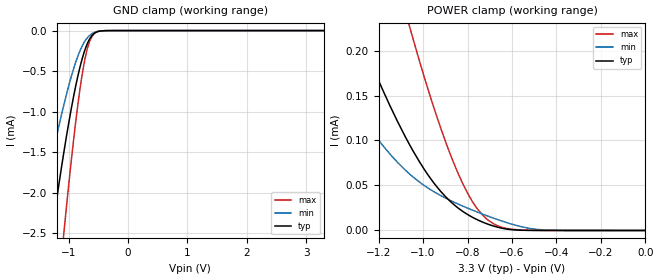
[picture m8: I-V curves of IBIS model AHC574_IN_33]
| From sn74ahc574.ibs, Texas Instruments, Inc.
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[Model]   AHC574_IN_33
Model_type  Input
Vinl = 0.9
Vinh = 2.1
| variable   typ   min   max
C_comp   1.37pF   0.98pF   1.70pF
[Temperature Range]   40   100   -40
| Ambient temperature   25   85   -40
[Voltage range]   3.3   3   3.6
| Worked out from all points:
|   GND clamp passes 1 mA (typ) near -0.97 V on its own axis
|   POWER clamp passes 1 mA (typ) near -2.27 V on its own axis
[GND Clamp]
| AHC574_IN_33
|   Voltage   I(typ)   I(min)   I(max)
-3.3V     -17mA      -11.03mA   -23.02mA
-1.53V    -3.897mA   -2.48mA    -6.164mA
-1.29V    -2.531mA   -1.59mA    -4.125mA
-1.255V   -2.347mA   -1.47mA    -3.84mA
-1.105V   -1.604mA   -983.1uA   -2.663mA
-1.075V   -1.466mA   -892.6uA   -2.438mA
-910mV    -781.9uA   -451.4uA   -1.295mA
-775mV    -351.6uA   -192.7uA   -547.4uA
-680mV    -149.8uA   -83.75uA   -205.8uA
-580mV    -40.35uA   -26.33uA   -44.58uA
-380mV    -1.07uA    -806.4nA   -548.9nA
3.3V      2.685nA    5.487nA    12.92nA
[POWER Clamp]
| AHC574_IN_33
|   Voltage   I(typ)   I(min)   I(max)
-3.3V     2.071mA    1.373mA    3.367mA
-1.505V   363.5uA    222.8uA    695.4uA
-1.295V   223uA      133.8uA    457.6uA
-1.185V   158.2uA    95.72uA    343.9uA
-1.06V    95.09uA    62.63uA    226.2uA
-965mV    57.34uA    45.17uA    147uA
-865mV    29.57uA    31.94uA    76.87uA
-795mV    17.05uA    24.36uA    39.35uA
-720mV    8.096uA    17.05uA    14.18uA
-600mV    847.3nA    6.953uA    1.319uA
-450mV    14.5nA     452nA      64.29nA
-48.03fV  2.685nA    409.8pA    20.12nA
